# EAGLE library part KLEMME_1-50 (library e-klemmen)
Klemme 50 Pol.
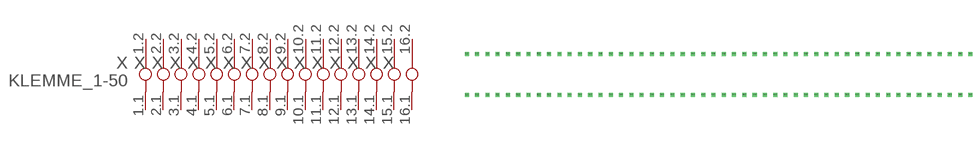
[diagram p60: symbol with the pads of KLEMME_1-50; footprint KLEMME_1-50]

Designator prefix X; gates 1=KLEMME_1-1 2=KLEMME_2 3=KLEMME_3 4=KLEMME_4 5=KLEMME_5 6=KLEMME_6 7=KLEMME_7 8=KLEMME_8 9=KLEMME_9 10=KLEMME_10 11=KLEMME_11 12=KLEMME_12 13=KLEMME_13 14=KLEMME_14 15=KLEMME_15 16=KLEMME_16 17=KLEMME_17 18=KLEMME_18 19=KLEMME_19 20=KLEMME_20 21=KLEMME_21 22=KLEMME_22 23=KLEMME_23 24=KLEMME_24 25=KLEMME_25 26=KLEMME_26 27=KLEMME_27 28=KLEMME_28 29=KLEMME_29 30=KLEMME_30 31=KLEMME_31 32=KLEMME_32 33=KLEMME_33 34=KLEMME_34 35=KLEMME_35 36=KLEMME_36 37=KLEMME_37 38=KLEMME_38 39=KLEMME_39 40=KLEMME_40 41=KLEMME_41 42=KLEMME_42 43=KLEMME_43 44=KLEMME_44 45=KLEMME_45 46=KLEMME_46 47=KLEMME_47 48=KLEMME_48 49=KLEMME_49 50=KLEMME_50

## KLEMME_1-50  [KLEMME_1-50]
1.1  1:1.1  pas
1.2  1:1.2  pas
2.1  2:2.1  pas
2.2  2:2.2  pas
3.1  3:3.1  pas
3.2  3:3.2  pas
4.1  4:4.1  pas
4.2  4:4.2  pas
5.1  5:5.1  pas
5.2  5:5.2  pas
6.1  6:6.1  pas
6.2  6:6.2  pas
7.1  7:7.1  pas
7.2  7:7.2  pas
8.1  8:8.1  pas
8.2  8:8.2  pas
9.1  9:9.1  pas
9.2  9:9.2  pas
10.1  10:10.1  pas
10.2  10:10.2  pas
11.1  11:11.1  pas
11.2  11:11.2  pas
12.1  12:12.1  pas
12.2  12:12.2  pas
13.1  13:13.1  pas
13.2  13:13.2  pas
14.1  14:14.1  pas
14.2  14:14.2  pas
15.1  15:15.1  pas
15.2  15:15.2  pas
16.1  16:16.1  pas
16.2  16:16.2  pas
17.1  17:17.1  pas
17.2  17:17.2  pas
18.1  18:18.1  pas
18.2  18:18.2  pas
19.1  19:19.1  pas
19.2  19:19.2  pas
20.1  20:20.1  pas
20.2  20:20.2  pas
21.1  21:21.1  pas
21.2  21:21.2  pas
22.1  22:22.1  pas
22.2  22:22.2  pas
23.1  23:23.1  pas
23.2  23:23.2  pas
24.1  24:24.1  pas
24.2  24:24.2  pas
25.1  25:25.1  pas
25.2  25:25.2  pas
26.1  26:26.1  pas
26.2  26:26.2  pas
27.1  27:27.1  pas
27.2  27:27.2  pas
28.1  28:28.1  pas
28.2  28:28.2  pas
29.1  29:29.1  pas
29.2  29:29.2  pas
30.1  30:30.1  pas
30.2  30:30.2  pas
31.1  31:31.1  pas
31.2  31:31.2  pas
32.1  32:32.1  pas
32.2  32:32.2  pas
33.1  33:33.1  pas
33.2  33:33.2  pas
34.1  34:34.1  pas
34.2  34:34.2  pas
35.1  35:35.1  pas
35.2  35:35.2  pas
36.1  36:36.1  pas
36.2  36:36.2  pas
37.1  37:37.1  pas
37.2  37:37.2  pas
38.1  38:38.1  pas
38.2  38:38.2  pas
39.1  39:39.1  pas
39.2  39:39.2  pas
40.1  40:40.1  pas
40.2  40:40.2  pas
41.1  41:41.1  pas
41.2  41:41.2  pas
42.1  42:42.1  pas
42.2  42:42.2  pas
43.1  43:43.1  pas
43.2  43:43.2  pas
44.1  44:44.1  pas
44.2  44:44.2  pas
45.1  45:45.1  pas
45.2  45:45.2  pas
46.1  46:46.1  pas
46.2  46:46.2  pas
47.1  47:47.1  pas
47.2  47:47.2  pas
48.1  48:48.1  pas
48.2  48:48.2  pas
49.1  49:49.1  pas
49.2  49:49.2  pas
50.1  50:50.1  pas
50.2  50:50.2  pas

## Footprint KLEMME_1-50 (pad centres in mm)
Dummy
drill 0.5 pad 1 square: 1.1 0,-12.7; 1.2 0,-2.54; 2.1 2.54,-12.7; 2.2 2.54,-2.54; 3.1 5.08,-12.7; 3.2 5.08,-2.54; 4.1 7.62,-12.7; 4.2 7.62,-2.54; 5.1 10.16,-12.7; 5.2 10.16,-2.54; 6.1 12.7,-12.7; 6.2 12.7,-2.54; 7.1 15.24,-12.7; 7.2 15.24,-2.54; 8.1 17.78,-12.7; 8.2 17.78,-2.54; 9.1 20.32,-12.7; 9.2 20.32,-2.54; 10.1 22.86,-12.7; 10.2 22.86,-2.54; 11.1 25.4,-12.7; 11.2 25.4,-2.54; 12.1 27.94,-12.7; 12.2 27.94,-2.54; 13.1 30.48,-12.7; 13.2 30.48,-2.54; 14.1 33.02,-12.7; 14.2 33.02,-2.54; 15.1 35.56,-12.7; 15.2 35.56,-2.54; 16.1 38.1,-12.7; 16.2 38.1,-2.54; 17.1 40.64,-12.7; 17.2 40.64,-2.54; 18.1 43.18,-12.7; 18.2 43.18,-2.54; 19.1 45.72,-12.7; 19.2 45.72,-2.54; 20.1 48.26,-12.7; 20.2 48.26,-2.54; 21.1 50.8,-12.7; 21.2 50.8,-2.54; 22.1 53.34,-12.7; 22.2 53.34,-2.54; 23.1 55.88,-12.7; 23.2 55.88,-2.54; 24.1 58.42,-12.7; 24.2 58.42,-2.54; 25.1 60.96,-12.7; 25.2 60.96,-2.54; 26.1 63.5,-12.7; 26.2 63.5,-2.54; 27.1 66.04,-12.7; 27.2 66.04,-2.54; 28.1 68.58,-12.7; 28.2 68.58,-2.54; 29.1 71.12,-12.7; 29.2 71.12,-2.54; 30.1 73.66,-12.7; 30.2 73.66,-2.54; 31.1 76.2,-12.7; 31.2 76.2,-2.54; 32.1 78.74,-12.7; 32.2 78.74,-2.54; 33.1 81.28,-12.7; 33.2 81.28,-2.54; 34.1 83.82,-12.7; 34.2 83.82,-2.54; 35.1 86.36,-12.7; 35.2 86.36,-2.54; 36.1 88.9,-12.7; 36.2 88.9,-2.54; 37.1 91.44,-12.7; 37.2 91.44,-2.54; 38.1 93.98,-12.7; 38.2 93.98,-2.54; 39.1 96.52,-12.7; 39.2 96.52,-2.54; 40.1 99.06,-12.7; 40.2 99.06,-2.54; 41.1 101.6,-12.7; 41.2 101.6,-2.54; 42.1 104.14,-12.7; 42.2 104.14,-2.54; 43.1 106.68,-12.7; 43.2 106.68,-2.54; 44.1 109.22,-12.7; 44.2 109.22,-2.54; 45.1 111.76,-12.7; 45.2 111.76,-2.54; 46.1 114.3,-12.7; 46.2 114.3,-2.54; 47.1 116.84,-12.7; 47.2 116.84,-2.54; 48.1 119.38,-12.7; 48.2 119.38,-2.54; 49.1 121.92,-12.7; 49.2 121.92,-2.54; 50.1 124.46,-12.7; 50.2 124.46,-2.54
